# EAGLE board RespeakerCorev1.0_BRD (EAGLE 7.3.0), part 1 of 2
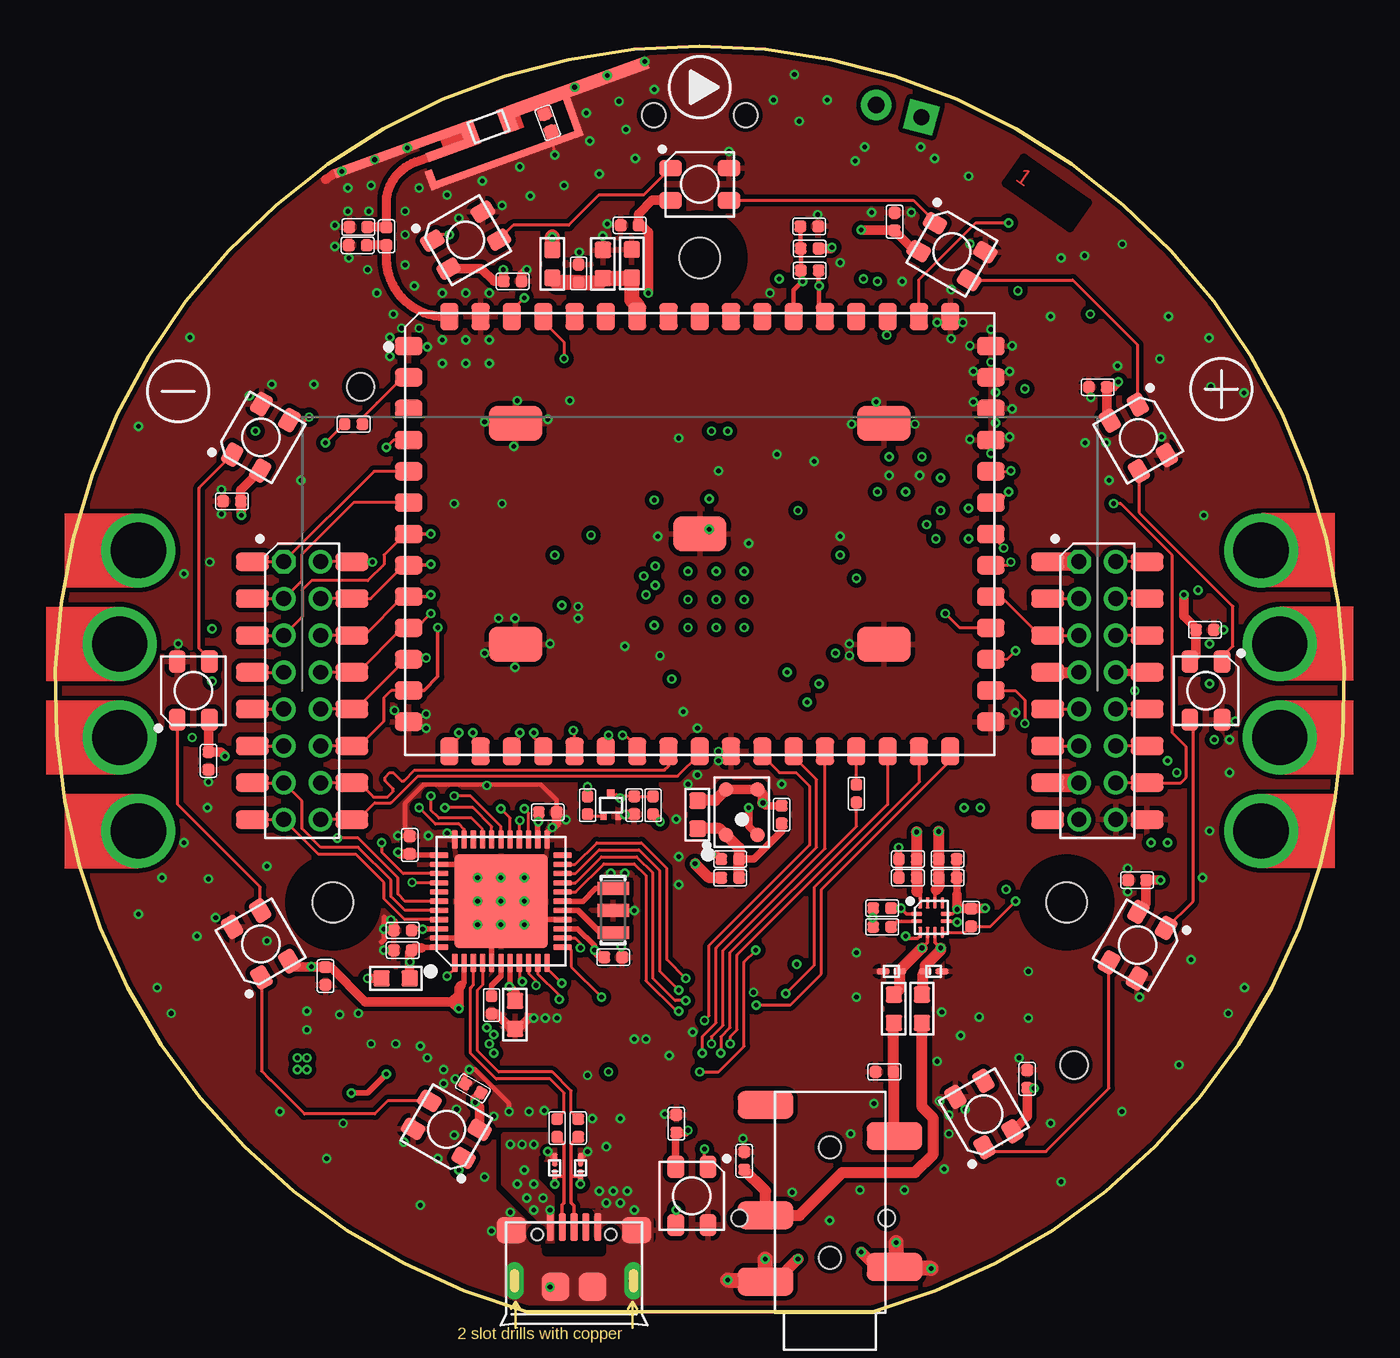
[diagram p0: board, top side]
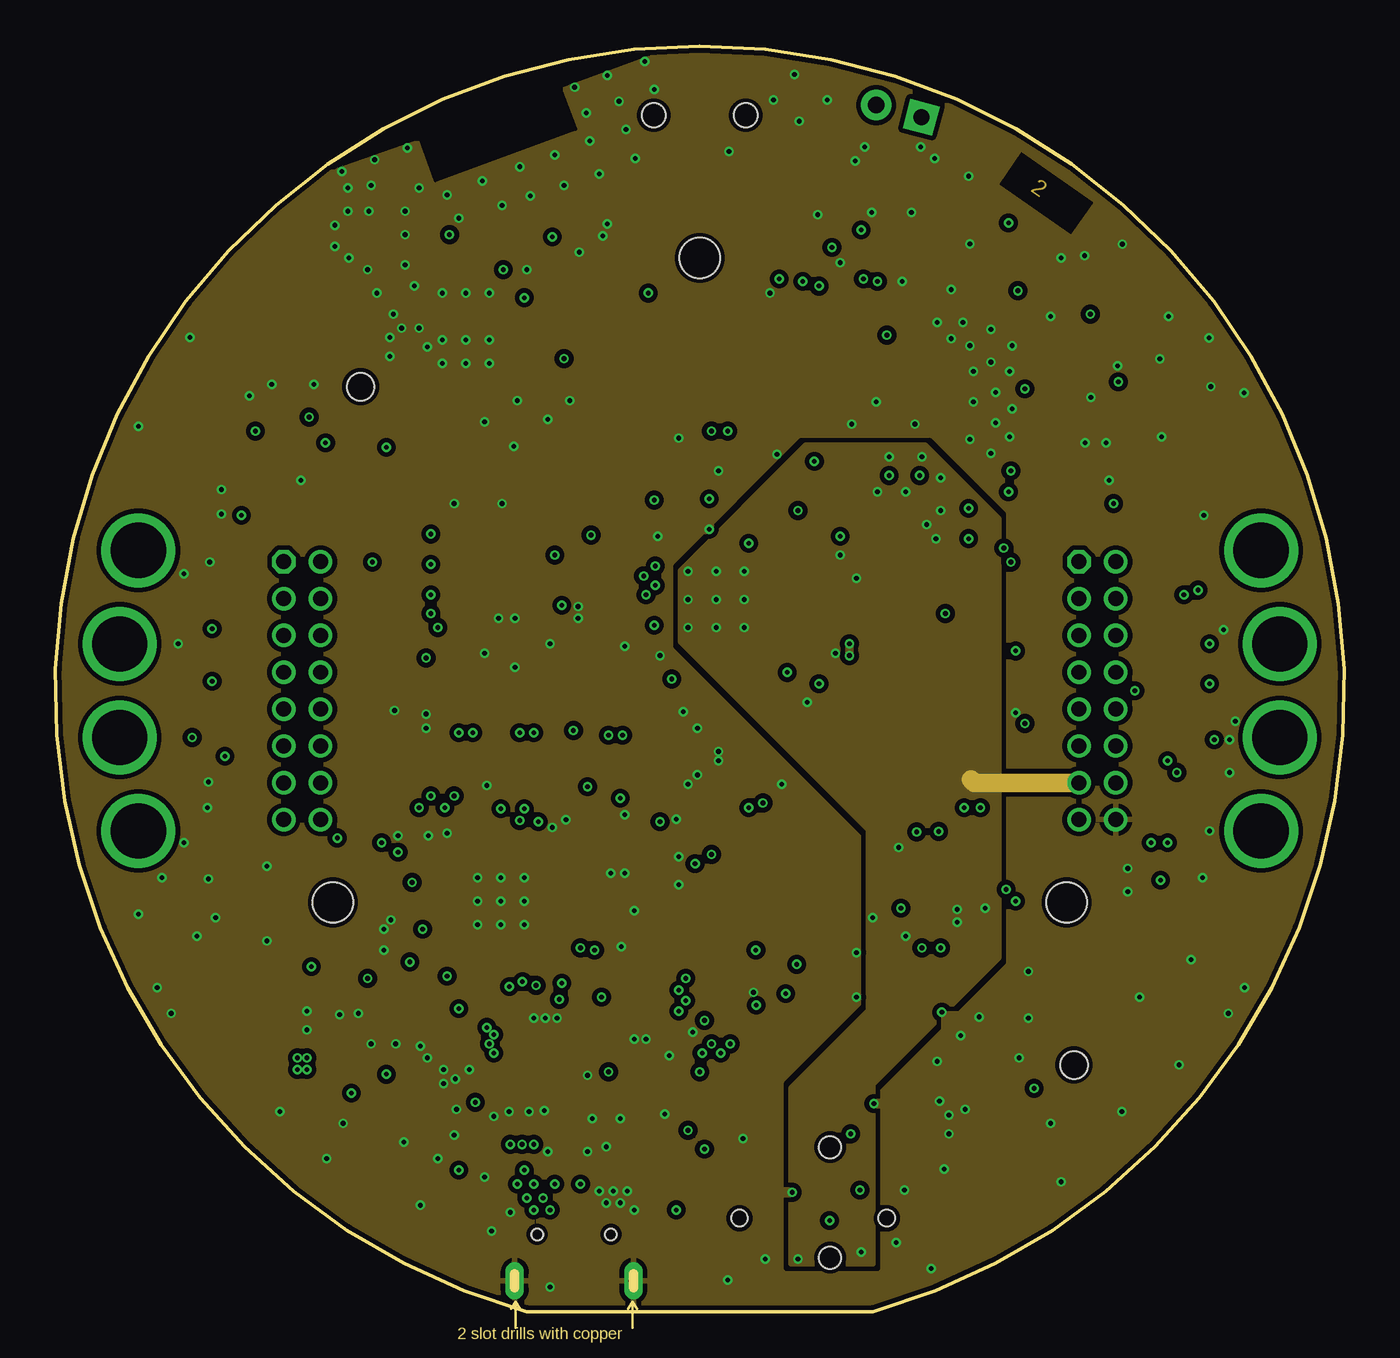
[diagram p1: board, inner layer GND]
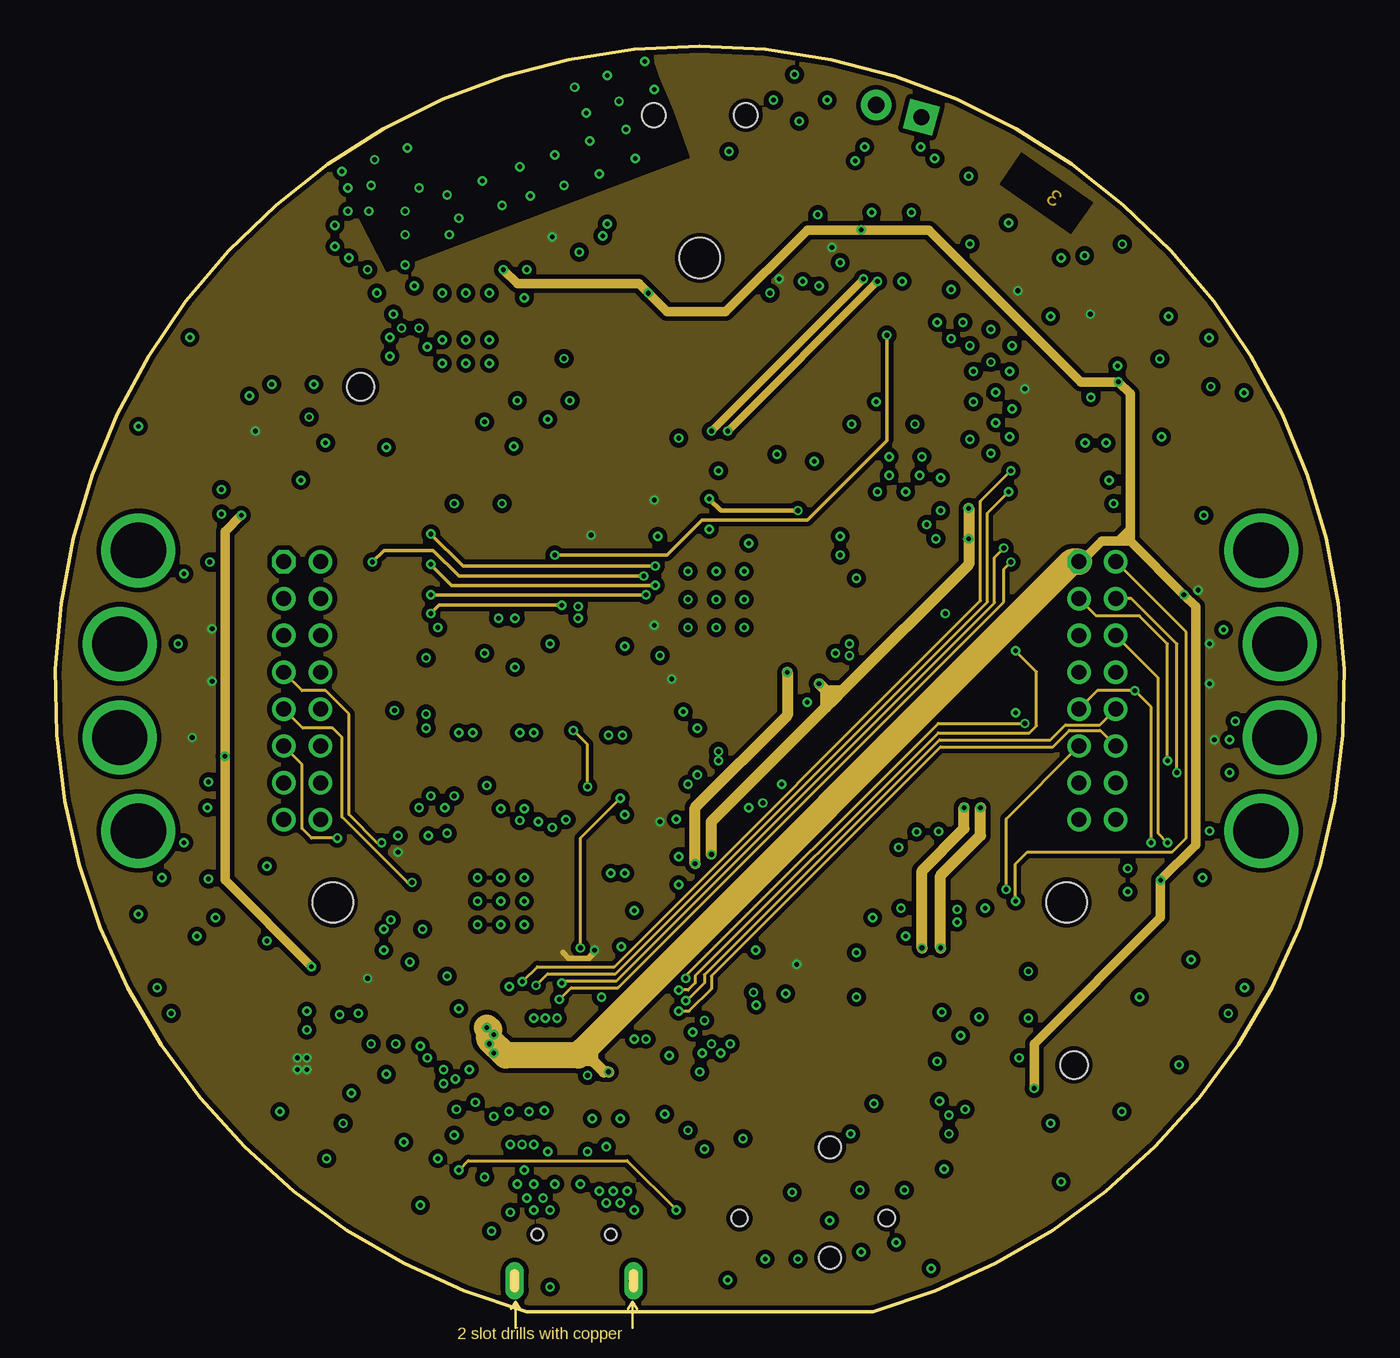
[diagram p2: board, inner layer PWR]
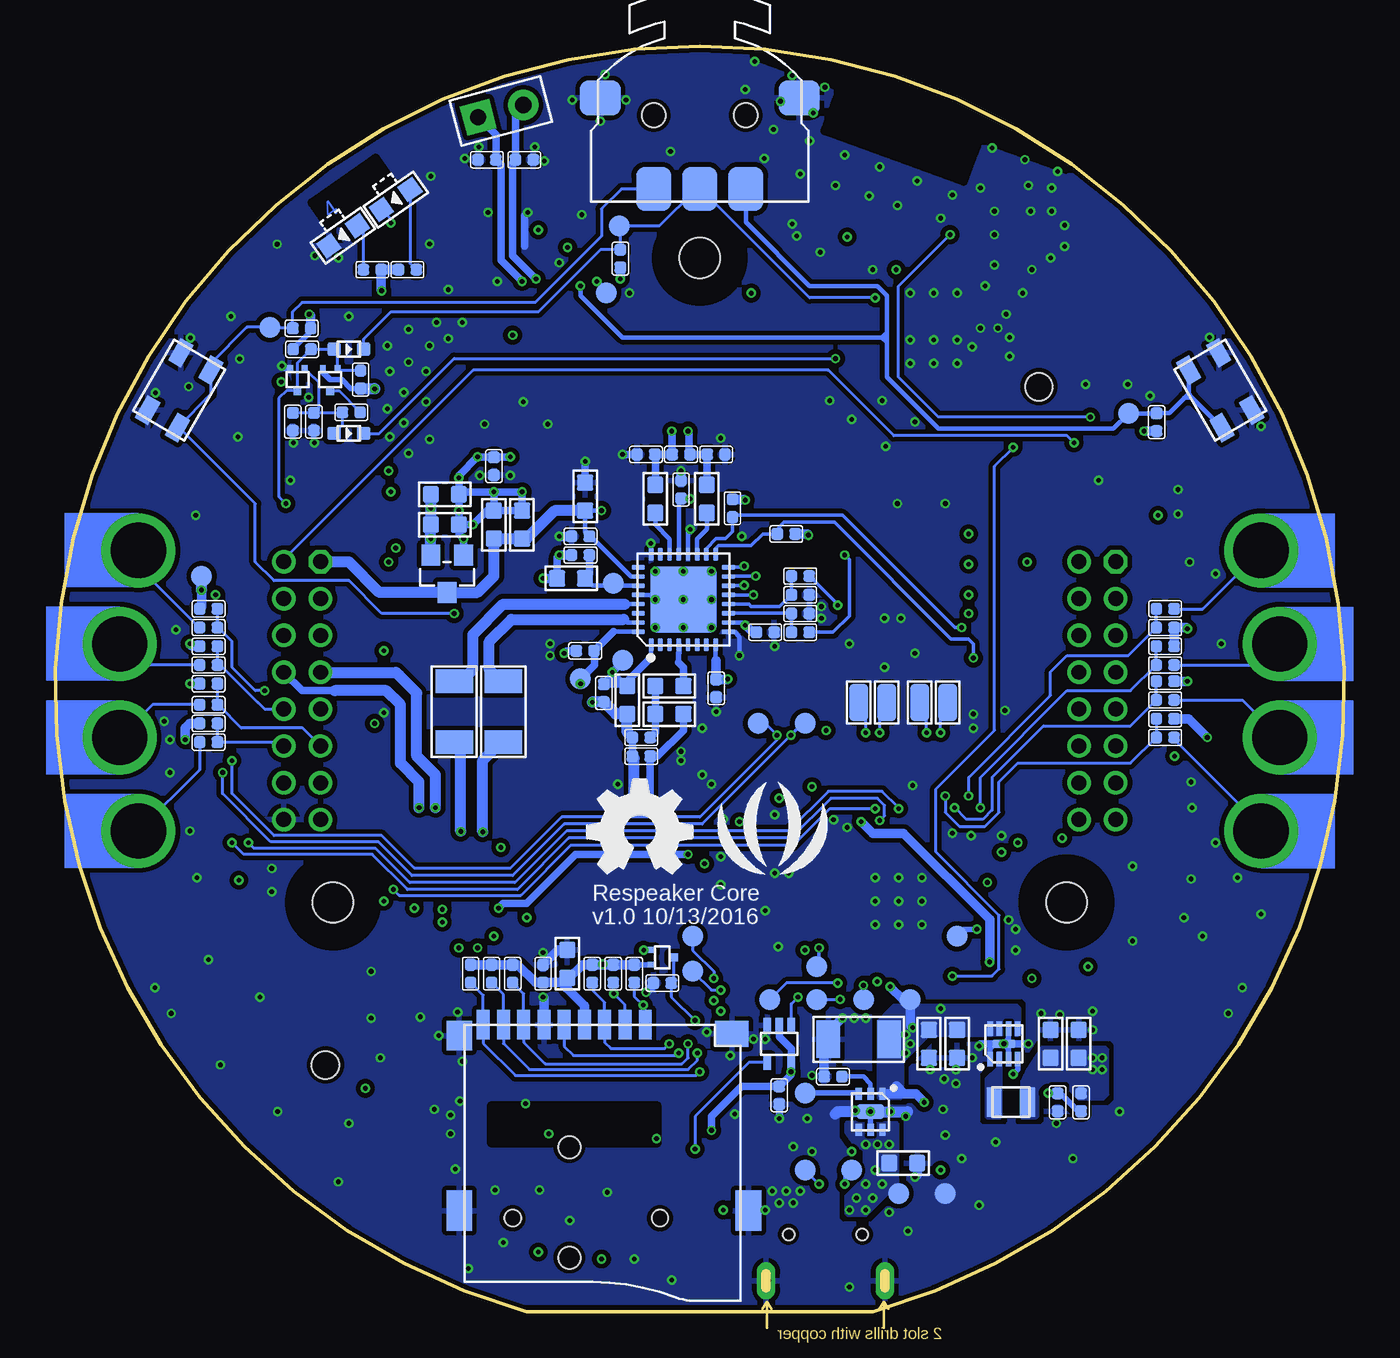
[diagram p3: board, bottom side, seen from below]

Size 69.97 x 68.72 mm. Coordinates in mm from the lower left corner, seen from the top.
Outline: 25.59,0 44.38,0 arc329 25.59,0
Copper layers (1*2*15*16): Top 0.035mm / dielectric 0.2mm / GND 0.0175mm / dielectric 0.3mm / PWR 0.0175mm / dielectric 0.2mm / Bottom 0.035mm
Design rules "SeeedStudio_4layer_DRU_no_angle_20140221 *": minimum track width 1mil, minimum drill 10mil, track to track 6mil, track to pad 6mil, pad to pad 6mil, via to via 6mil, smd to smd 0mil, copper to edge 10mil, drill to drill 8mil, minimum pad ring 6mil, minimum via ring 4mil, stop-mask expansion 4mil, vias tented up to drill 25mil, thermal gap 10mil
Holes 2.2 mm at 15.07,22.22 34.98,57.22 54.9,22.22
Holes 1.5 mm at 16.57,50.23 55.3,13.4
tRestrict: area 32.6,54.9 to 37.3,59.6; area 12.7,19.9 to 17.4,24.6; area 52.6,19.9 to 57.3,24.6; area 51.6,58.9 to 56,62.6
bRestrict: area 32.6,54.9 to 37.3,59.6; area 12.7,19.9 to 17.4,24.6; area 52.6,19.9 to 57.3,24.6; area 51.6,58.9 to 56,62.6; area 17.8,10.7 to 18.2,11.9

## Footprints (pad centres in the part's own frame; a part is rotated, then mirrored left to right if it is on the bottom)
ANT2P-SMD-3.5X1.4MM-BOTTOM = smd 3 x 0.5: ANT -2.5,-0.45 | smd 0.72 x 0.4: C$1 2.8,-0.48; C$2 2.8,-1.32; P$3 2.8,-1.67 | smd 0.8 x 1.4: CHIP1 0.8,0; CHIP2 -1.4,0 | smd 8.4 x 0.4: G$1 0,-2 | smd 0.4 x 2.6: G$2 4.2,-0.9 | smd 0.4 x 1.1: G$4 -4.2,-1.65 | smd 8 x 0.7: GND1 5,0.35 | smd 8 x 0.5: GND2 -5,0.45
BUTTON3+2P-SMD-11.8X11.8X2.5MM = smd 1.9 x 2.4: 1 -2.5,0.7; 2 0,0.7; 3 2.5,0.7 | smd 2.2 x 1.9: 4 5.4,5.65; 5 -5.4,5.65 | hole 1.3: -2.5,4.7; 2.5,4.7
C0402 = smd 0.635 x 0.635: 1 0,0.484; 2 0,-0.484
C0603 = smd 0.889 x 0.889: 1 0,0.762; 2 0,-0.762
C1206 = smd 1.27 x 2.032: 1 -1.651,0; 2 1.651,0
LED4-SMD-3.5X3.7MM = smd 1.2 x 0.9: 1 -1.58,0.875; 2 -1.58,-0.875; 3 1.58,-0.875; 4 1.58,0.875
SOD-923 = smd 0.7 x 0.3: 1 -0.45,0; 2 0.45,0
LED-SIDE-VIEW-0603-RIGHT = smd 1 x 1: 1 0,-0.95; 2 0,0.95
SOD-523 = smd 0.762 x 0.7: + -0.8,0; - 0.8,0
L0603 = smd 0.889 x 0.889: 1 -0.762,0; 2 0.762,0
MICRO-USB5+4P-SMD-0.65-B = smd 0.381 x 1.524: 1 -1.3,-0.25; 2 -0.65,-0.25; 3 0,-0.25; 4 0.65,-0.25; 5 1.3,-0.25 | smd 1.6 x 1.397: S1 -3.4,-0.427; S6 3.4,-0.427 | drill 0.508 pad 1.016 long: S2 -3.226,-3.175; S5 3.226,-3.175 | smd 1.5 x 1.5: S3 -1,-3.5; S4 1,-3.5 | hole 0.635: -2,-0.65; 2,-0.65
AUDIO5P-14X5X4.4MM = smd 3 x 1.5: 2 -3.5,-11.6; 3 -3.5,-4.5; 4 3.5,-3.7; 5 3.5,-7.3; 6 3.5,-13.3 | hole 1.2: 0,-5; 0,-11
1P-DIP-6X4MM = drill 3 pad 4: 1 0,0
H2-2.54 = drill 0.889 pad 1.651 square: 1 0,1.27 | drill 0.889 pad 1.651: 2 0,-1.27
H2X8-SMD_DRILL-2.0 = smd 1.8 x 1: 1 -2.7,7; 2 2.7,7; 3 -2.7,5; 4 2.7,5; 5 -2.7,3; 6 2.7,3; 7 -2.7,1; 8 2.7,1; 9 -2.7,-1; 10 2.7,-1; 11 -2.7,-3; 12 2.7,-3; 13 -2.7,-5; 14 2.7,-5; 15 -2.7,-7; 16 2.7,-7 | drill 0.813 pad 1.27 octagon: P$1 -1,7 | drill 0.813 pad 1.27: P$2 1,7; P$3 -1,5; P$4 1,5; P$5 -1,3; P$6 1,3; P$7 -1,1; P$8 1,1; P$9 -1,-1; P$10 1,-1; P$11 -1,-3; P$12 1,-3; P$13 -1,-5; P$14 1,-5; P$15 -1,-7; P$16 1,-7
MICRO-SD9+4P-SMD-16.1X14.5X1.85MM = smd 1.6 x 0.7: 1 0,2.25; 2 0,1.15; 3 0,0.05; 4 0,-1.05; 5 0,-2.15; 6 0,-3.25; 7 0,-4.35; 8 0,-5.45; 9 0,-6.55 | smd 1.6 x 1.4: G1 0.6,-7.85 | smd 2.2 x 1.4: G2 10.1,-7.85; G3 10.1,7.85 | smd 1.4 x 1.8: G4 0.5,6.95 | hole 0.9: 10.5,-4.95; 10.5,3.05
SW4P-SMD-4.5X3.2X2.5MM = smd 1.4 x 0.8: 1 -1.8,-0.94; 2 1.8,-0.94; 3 1.8,0.94; 4 -1.8,0.94
L201610 = smd 0.8 x 1.6: 1 -0.9,0; 2 0.9,0
R0402 = smd 0.635 x 0.635: 1 0,0.484; 2 0,-0.484
MIC4-SMD-3.76X2.95MM = smd 0.8 x 0.8: 1 0.85,1.23; 2 0.85,-1.23; 3 -0.85,-1.23; 4 -0.85,1.23
SOT-723 = smd 0.32 x 0.4: 1 -0.4,-0.6; 2 0.4,-0.6 | smd 0.42 x 0.5: 3 0,0.6
TP-D45MIL = smd 1.143 x 1.143: T 0,0
TP-80X40MIL = smd 2.032 x 1.016: 1 0,0
DFN6G-0.65-2X2MM = smd 0.65 x 0.35: 1 -0.975,0.65; 2 -0.975,0; 3 -0.975,-0.65; 4 0.975,-0.65; 5 0.975,0; 6 0.975,0.65 | smd 0.8 x 1.5: PAD 0,0
DFN8G-0.5-2X2MM = smd 0.8 x 0.3: 1 -0.827,0.75; 2 -0.827,0.25; 3 -0.827,-0.25; 4 -0.827,-0.75; 5 0.827,-0.75; 6 0.827,-0.25; 7 0.827,0.25; 8 0.827,0.75 | smd 0.45 x 1.3: 9 0,0
SOT-353 = smd 0.4 x 0.8: 1 -0.65,-1; 2 0,-1; 3 0.65,-1; 4 0.65,1; 5 -0.65,1
SOT-23 = smd 1.016 x 1.143: 1 -0.889,-1.016; 2 0.889,-1.016; 3 0,1.016
QFN32G-0.5-5X5MM = smd 0.7 x 0.25: 1 -2.45,1.75; 2 -2.45,1.25; 3 -2.45,0.75; 4 -2.45,0.25; 5 -2.45,-0.25; 6 -2.45,-0.75; 7 -2.45,-1.25; 8 -2.45,-1.75; 17 2.45,-1.75; 18 2.45,-1.25; 19 2.45,-0.75; 20 2.45,-0.25; 21 2.45,0.25; 22 2.45,0.75; 23 2.45,1.25; 24 2.45,1.75 | smd 0.25 x 0.7: 9 -1.75,-2.45; 10 -1.25,-2.45; 11 -0.75,-2.45; 12 -0.25,-2.45; 13 0.25,-2.45; 14 0.75,-2.45; 15 1.25,-2.45; 16 1.75,-2.45; 25 1.75,2.45; 26 1.25,2.45; 27 0.75,2.45; 28 0.25,2.45; 29 -0.25,2.45; 30 -0.75,2.45; 31 -1.25,2.45; 32 -1.75,2.45 | smd 3.6 x 3.6: 33 0,0
LGA65-1.7-24X32X1.8MM = smd 1.5 x 1: 1 -15.8,10.2; 2 -15.8,8.5; 3 -15.8,6.8; 4 -15.8,5.1; 5 -15.8,3.4; 6 -15.8,1.7; 7 -15.8,0; 8 -15.8,-1.7; 9 -15.8,-3.4; 10 -15.8,-5.1; 11 -15.8,-6.8; 12 -15.8,-8.5; 13 -15.8,-10.2; 31 15.8,-10.2; 32 15.8,-8.5; 33 15.8,-6.8; 34 15.8,-5.1; 35 15.8,-3.4; 36 15.8,-1.7; 37 15.8,0; 38 15.8,1.7; 39 15.8,3.4; 40 15.8,5.1; 41 15.8,6.8; 42 15.8,8.5; 43 15.8,10.2 | smd 1 x 1.5: 14 -13.6,-11.8; 15 -11.9,-11.8; 16 -10.2,-11.8; 17 -8.5,-11.8; 18 -6.8,-11.8; 19 -5.1,-11.8; 20 -3.4,-11.8; 21 -1.7,-11.8; 22 0,-11.8; 23 1.7,-11.8; 24 3.4,-11.8; 25 5.1,-11.8; 26 6.8,-11.8; 27 8.5,-11.8; 28 10.2,-11.8; 29 11.9,-11.8; 30 13.6,-11.8; 44 13.6,11.8; 45 11.9,11.8; 46 10.2,11.8; 47 8.5,11.8; 48 6.8,11.8; 49 5.1,11.8; 50 3.4,11.8; 51 1.7,11.8; 52 0,11.8; 53 -1.7,11.8; 54 -3.4,11.8; 55 -5.1,11.8; 56 -6.8,11.8; 57 -8.5,11.8; 58 -10.2,11.8; 59 -11.9,11.8; 60 -13.6,11.8 | smd 2.9 x 1.9: 61 10,6; 62 -10,6; 63 -10,-6; 64 10,-6; 65 0,0
VQFN-44 = smd 1 x 0.3: 1 -3.35,2.5; 2 -3.35,2; 3 -3.35,1.5; 4 -3.35,1; 5 -3.35,0.5; 6 -3.35,0; 7 -3.35,-0.5; 8 -3.35,-1; 9 -3.35,-1.5; 10 -3.35,-2; 11 -3.35,-2.5; 23 3.35,-2.5; 24 3.35,-2; 25 3.35,-1.5; 26 3.35,-1; 27 3.35,-0.5; 28 3.35,0; 29 3.35,0.5; 30 3.35,1; 31 3.35,1.5; 32 3.35,2; 33 3.35,2.5 | smd 0.3 x 1: 12 -2.5,-3.35; 13 -2,-3.35; 14 -1.5,-3.35; 15 -1,-3.35; 16 -0.5,-3.35; 17 0,-3.35; 18 0.5,-3.35; 19 1,-3.35; 20 1.5,-3.35; 21 2,-3.35; 22 2.5,-3.35; 34 2.5,3.35; 35 2,3.35; 36 1.5,3.35; 37 1,3.35; 38 0.5,3.35; 39 0,3.35; 40 -0.5,3.35; 41 -1,3.35; 42 -1.5,3.35; 43 -2,3.35; 44 -2.5,3.35 | smd 5.08 x 5.08: TAB 0,0
LEAD12P-SMD-0.4-1.8X1.8X0.5MM = smd 0.6 x 0.2: 1 -0.8,0.2; 2 -0.8,-0.2; 7 0.8,-0.2; 8 0.8,0.2 | smd 0.2 x 0.6: 3 -0.6,-0.8; 4 -0.2,-0.8; 5 0.2,-0.8; 6 0.6,-0.8; 9 0.6,0.8; 10 0.2,0.8; 11 -0.2,0.8; 12 -0.6,0.8
RESONATOR3-SMD-3.6X1.3X0.8MM = smd 0.7 x 1.7: 1 -1.2,0; 2 0,0; 3 1.2,0

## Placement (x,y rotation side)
ANT1  [ANT2P-SMD-3.5X1.4MM-BOTTOM]  23.8,64.45 20 top
BUTTON1  [BUTTON3+2P-SMD-11.8X11.8X2.5MM]  34.98,60.26 0 bottom
C1  100nF  [C0402]  45.56,59.19 0 top
C2  100nF  [C0402]  31.43,27.5 180 top
C3  100nF  [C0402]  56.59,50.2 90 top
C4  100nF  [C0402]  62.42,37.02 270 top
C5  10uF  [C0603]  23.94,8.06 270 bottom
C6  10uF  [C0603]  21.01,14.54 180 bottom
C7  10uF  [C0603]  22.54,14.54 180 bottom
C8  10uF  [C0603]  14.41,14.54 0 bottom
C9  10uF  [C0603]  15.93,14.54 0 bottom
C10  100uF 10V  [C1206]  26.35,14.8 0 bottom
C11  100nF  [C0402]  58.73,23.43 90 top
C12  100nF  [C0402]  52.76,12.64 0 top
C13  10uF  [C0603]  44.64,42.74 0 bottom
C14  10uF  [C0603]  46.16,42.74 0 bottom
C15  10uF  [C0603]  48.83,42.74 270 bottom
C16  10uF  [C0603]  48.83,44.39 270 bottom
C17  100nF  [C0402]  33.71,10.21 0 top
C18  10uF  [C0603]  34.86,26.99 0 top
C19  100nF  [C0402]  57.08,48.32 180 bottom
C20  33pF  [C0402]  29.52,38.93 270 bottom
C22  100nF  [C0402]  31.43,36.89 270 bottom
C23  100nF  [C0402]  34.1,33.85 180 bottom
C24  100nF  [C0402]  41.21,35.88 90 bottom
C25  100uF 10V  [C1206]  48.32,32.58 270 bottom
C26  100uF 10V  [C1206]  45.65,32.58 270 bottom
C27  100nF  [C0402]  53.4,50.61 0 bottom
C28  100pF  [C0402]  46.29,24.57 90 top
C29  100pF  [C0402]  48.45,24.57 270 top
C31  680nF DNP  [C0402]  36,46.55 90 bottom
C32  100pF  [C0402]  34.1,46.55 270 bottom
C33  100pF  [C0402]  37.91,46.55 90 bottom
C34  100pF  [C0402]  44.51,62.55 270 bottom
C35  100pF  [C0402]  46.54,62.55 90 bottom
C36  10uF  [C0603]  36.64,33.97 90 bottom
C37  100nF  [C0402]  39.43,26.99 0 top
C38  33pF  [C0402]  38.16,30.16 90 bottom
C39  33pF  [C0402]  38.16,31.18 90 bottom
C41  100nF  [C0402]  22.67,12.13 60 top
C42  100nF  [C0402]  14.66,18.22 180 top
C43  100nF  [C0402]  8.31,29.91 180 top
C44  100nF  [C0402]  9.58,44.01 90 top
C45  100nF  [C0402]  24.82,55.94 270 top
C46  100nF  [C0402]  31.17,58.99 90 top
C48  100nF  [C0402]  30.67,11.75 180 bottom
C49  10uF  [C0603]  41.21,44.26 180 bottom
C50  100nF  [C0402]  36,44.64 0 bottom
C51  100nF  [C0402]  41.46,42.1 90 bottom
C52  10uF  [C0603]  38.92,33.21 0 bottom
C53  100nF  [C0402]  40.19,33.59 180 bottom
C54  10uF  [C0603]  41.97,39.81 270 bottom
C55  100nF  [C0402]  41.46,41.08 90 bottom
C56  10uF  [C0603]  42.18,18.88 180 bottom
C57  1uF  [C0402]  43.49,18.35 180 bottom
C58  10uF  [C0603]  29.73,56.88 180 top
C59  10uF  [C0603]  31.29,56.91 180 top
C60  100nF  [C0402]  28.41,56.37 0 top
C61  1uF  [C0402]  40.93,58.93 270 top
C62  1uF  [C0402]  23.68,16.65 180 top
C63  100nF  [C0402]  30.29,19.24 270 top
C64  100nF  [C0402]  19.24,25.34 0 top
C65  100nF  [C0402]  26.73,27.11 270 top
C66  100nF  [C0402]  18.86,19.62 90 top
C67  100nF  [C0402]  18.86,20.7 90 top
C68  100nF  [C0402]  44.89,20.89 90 top
C69  100nF  [C0402]  44.89,21.91 90 top
C71  33pF  [C0402]  37.4,8.19 0 top
C72  33pF  [C0402]  45.02,13.02 90 top
C74  10uF  [C0603]  24.95,16.12 0 top
C75  33pF  [C0402]  29.52,37.91 270 bottom
D1  SK6812  [LED4-SMD-3.5X3.7MM]  48.68,57.56 150 top
D2  SK6812  [LED4-SMD-3.5X3.7MM]  58.8,47.45 120 top
D3  SK6812  [LED4-SMD-3.5X3.7MM]  62.47,33.72 90 top
D4  SK6812  [LED4-SMD-3.5X3.7MM]  58.76,19.9 60 top
D5  SK6812  [LED4-SMD-3.5X3.7MM]  50.42,10.73 300 top
D6  DF2S6.8FS  [SOD-923]  28.51,7.81 90 top
D7  DF2S6.8FS  [SOD-923]  27.11,7.81 90 top
D8  SK6812  [LED4-SMD-3.5X3.7MM]  34.55,6.29 90 top
D9  SK6812  [LED4-SMD-3.5X3.7MM]  21.23,9.9 330 top
D10  SK6812  [LED4-SMD-3.5X3.7MM]  11.15,19.96 300 top
D11  Green  [LED-SIDE-VIEW-0603-RIGHT]  54.35,58.42 125 bottom
D12  Red  [LED-SIDE-VIEW-0603-RIGHT]  51.49,60.39 125 bottom
D13  SK6812  [LED4-SMD-3.5X3.7MM]  7.49,33.72 270 top
D14  SK6812  [LED4-SMD-3.5X3.7MM]  11.15,47.47 240 top
D15  DF2S6.8FS  [SOD-923]  45.4,18.48 180 top
D16  DF2S6.8FS  [SOD-923]  47.68,18.48 0 top
D18  SK6812  [LED4-SMD-3.5X3.7MM]  22.27,58.19 210 top
D19  SK6812  [LED4-SMD-3.5X3.7MM]  34.98,61.22 180 top
D20  1N4148WT  [SOD-523]  54.03,52.26 0 bottom
D21  1N4148WT  [SOD-523]  54.03,47.69 0 bottom
FB1  120R 500mA  [L0603]  26.98,56.9 270 top
FB2  120R-500mA  [L0603]  18.47,18.1 0 top
FR1  [SEEEDSTUDIO-PCB-FRAME]  not placed on the board
FR2  [SEEEDSTUDIO-PCB-FRAME]  not placed on the board
FR3  [SEEEDSTUDIO-PCB-FRAME]  not placed on the board
FR4  [SEEEDSTUDIO-PCB-FRAME]  not placed on the board
FR5  [SEEEDSTUDIO-PCB-FRAME]  not placed on the board
FR7  [SEEEDSTUDIO-PCB-FRAME]  not placed on the board
J1  MICRO-USB  [MICRO-USB5+4P-SMD-0.65-B]  28.16,4.85 0 top
J2  PJ327-327  [AUDIO5P-14X5X4.4MM]  42.06,-2.07 180 top
J3  [1P-DIP-6X4MM]  65.46,41.34 90 top
J4  DNP  [H2-2.54]  45.79,65.19 105 bottom
J5  EH  [H2X8-SMD_DRILL-2.0]  13.39,33.72 0 top
J6  [H2X8-SMD_DRILL-2.0]  56.57,33.72 0 top
J7  [MICRO-SD9+4P-SMD-16.1X14.5X1.85MM]  40.19,15.58 270 bottom
J8  [1P-DIP-6X4MM]  66.48,36.26 90 top
J9  [1P-DIP-6X4MM]  66.48,31.18 90 top
J10  [1P-DIP-6X4MM]  65.46,26.1 90 top
J11  [1P-DIP-6X4MM]  4.5,26.1 270 top
J12  [1P-DIP-6X4MM]  3.49,31.18 270 top
J13  [1P-DIP-6X4MM]  3.49,36.26 270 top
J14  [1P-DIP-6X4MM]  4.5,41.34 270 top
K1  [SW4P-SMD-4.5X3.2X2.5MM]  6.72,50.04 300 bottom
K2  [SW4P-SMD-4.5X3.2X2.5MM]  63.25,50.04 60 bottom
L1  0.47uH  [L201610]  18.09,11.37 0 bottom
L2  BLM18BD252SN1  [L0603]  47.05,16.45 270 top
L4  BLM18BD252SN1  [L0603]  45.53,16.45 270 top
L6  BLM18BD252SN1  [L0603]  37.4,44.13 90 bottom
L7  BLM18BD252SN1  [L0603]  34.6,44.13 90 bottom
L8  BLM18BD252SN1  [L0603]  36.64,32.45 180 bottom
LC1  6.8nH  [R0402]  16.45,58.89 90 top
LC2  1.5pF  [R0402]  16.41,57.9 90 top
LC3  1.6pF  [R0402]  17.98,58.4 0 top
LC4  dnp  [R0402]  26.73,64.55 20 top
MIC1  SAO-3729-M-42-008  [MIC4-SMD-3.76X2.95MM]  37.27,27.11 180 top
Q1  CJ3134K  [SOT-723]  30.16,27.5 0 top
Q2  CJ3139K  [SOT-723]  37.02,19.24 270 bottom
Q3  CJ3139K  [SOT-723]  55.05,50.61 180 bottom
Q4  CJ3134K  [SOT-723]  56.83,50.61 180 bottom
R1  10k  [R0402]  32.44,27.5 0 top
R2  1k  [R0402]  28.89,27.5 180 top
R3  100k_1%  [R0402]  55.94,48.32 0 bottom
R4  10k dnp  [R0402]  56.57,52.26 270 bottom
R5  100k_1%  [R0402]  14.28,11.37 180 bottom
R6  22K_1%  [R0402]  27.75,12.76 90 bottom
R7  22K_1%  [R0402]  15.55,11.37 180 bottom
R8  10M  [R0402]  61.65,31.94 270 bottom
R9  22R  [R0402]  27.24,9.97 0 top
R10  22R  [R0402]  28.38,9.97 0 top
R11  10k  [R0402]  39.29,57.18 0 bottom
R12  1k  [R0402]  52.76,56.58 90 bottom
R13  10M  [R0402]  9.71,32.19 90 bottom
R14  10M  [R0402]  9.71,34.23 90 bottom
R15  10M  [R0402]  9.71,36.13 90 bottom
R16  10M  [R0402]  9.71,37.15 90 bottom
R17  1k  [R0402]  50.86,56.58 270 bottom
R18  33R  [R0402]  9.71,38.16 90 bottom
R19  33R  [R0402]  61.65,30.92 270 bottom
R20  33R  [R0402]  9.71,35.12 90 bottom
R21  33R  [R0402]  9.71,33.21 90 bottom
R22  1k  [R0402]  10.18,48.3 0 bottom
R23  33R  [R0402]  9.71,31.18 90 bottom
R24  10k  [R0402]  47.43,18.35 180 bottom
R25  10k  [R0402]  46.29,18.35 180 bottom
R26  10k  [R0402]  45.14,18.35 180 bottom
R27  10k  [R0402]  40.83,18.35 180 bottom
R28  10k  [R0402]  39.68,18.35 180 bottom
R29  10k  [R0402]  38.54,18.35 180 bottom
R30  10k  [R0402]  46.29,23.56 90 top
R31  10k  [R0402]  48.45,23.56 270 top
R32  22R  [R0402]  43.49,28.13 180 top
R33  10k  [R0402]  56.6,53.4 90 bottom
R34  0R  [R0402]  46.16,45.91 180 bottom
R35  10M  [R0402]  61.65,34.1 270 bottom
R36  33R  [R0402]  61.65,32.96 270 bottom
R37  10M  [R0402]  61.65,36.13 270 bottom
R38  10k  [R0402]  33.21,43.62 180 bottom
R39  10k  [R0402]  30.29,42.23 90 bottom
R40  22R  [R0402]  29.52,39.94 90 bottom
R41  33R  [R0402]  61.65,35.12 270 bottom
R42  10M  [R0402]  61.65,38.16 270 bottom
R43  33R  [R0402]  61.65,37.15 270 bottom
R46  100k_1%  [R0402]  53.91,48.83 270 bottom
R47  2.2k  [R0402]  49.72,21.4 0 top
R48  0R  [R0402]  16.19,48.2 270 top
R49  22R  [R0402]  29.52,36.89 90 bottom
R53  10k  [R0402]  40.95,57.73 90 top
R55  0R DNP  [R0402]  40.96,56.53 90 top
R56  10k  [R0402]  37.02,17.84 90 bottom
R57  0R  [R0402]  36.64,23.56 90 top
R58  0R DNP  [R0402]  36.64,24.57 90 top
TP1  [TP-D45MIL]  23.55,16.95 180 bottom
TP2  [TP-D45MIL]  62.04,39.94 180 bottom
TP3  [TP-D45MIL]  24.19,6.41 180 bottom
TP4  [TP-D45MIL]  41.46,34.35 180 bottom
TP5  [TP-D45MIL]  26.09,16.95 270 bottom
TP6  [TP-D45MIL]  39.35,58.96 158 bottom
TP7  [TP-D45MIL]  28.63,16.95 270 bottom
TP8  [TP-D45MIL]  31.17,16.95 270 bottom
TP9  [TP-80X40MIL]  21.52,33.08 270 bottom
TP10  [TP-80X40MIL]  23.05,33.08 270 bottom
TP11  [TP-80X40MIL]  24.82,33.08 270 bottom
TP12  [TP-D45MIL]  11.69,48.77 60 bottom
TP13  [TP-D45MIL]  39.18,35.37 180 bottom
TP14  [TP-D45MIL]  39.68,39.56 180 bottom
TP15  [TP-D45MIL]  58.33,53.45 188 bottom
TP16  [TP-D45MIL]  29.27,31.94 180 bottom
TP17  [TP-D45MIL]  31.81,31.94 180 bottom
TP18  [TP-D45MIL]  21.65,6.41 0 bottom
TP19  [TP-D45MIL]  26.73,7.68 0 bottom
TP20  [TP-D45MIL]  29.27,7.68 0 bottom
TP21  [TP-D45MIL]  29.27,11.87 0 bottom
TP22  [TP-80X40MIL]  26.35,33.08 270 bottom
TP23  [TP-D45MIL]  28.63,18.73 0 bottom
TP24  [TP-D45MIL]  35.37,18.48 180 bottom
TP25  [TP-D45MIL]  35.37,20.38 180 bottom
TP26  [TP-D45MIL]  40.06,55.31 0 bottom
TP27  [TP-D45MIL]  21.01,20.38 0 bottom
U1  ETA6020  [DFN6G-0.65-2X2MM]  25.71,10.86 270 bottom
U2  ETA3410  [DFN8G-0.5-2X2MM]  18.47,14.54 90 bottom
U3  74HC1G08  [SOT-353]  30.67,14.54 180 bottom
U4  AP7333  [SOT-23]  48.7,40.07 180 bottom
U5  WM8960  [QFN32G-0.5-5X5MM]  35.87,38.67 90 bottom
U6  AI7688H  [LGA65-1.7-24X32X1.8MM]  34.98,42.23 0 top
U7  ATMEGA32U4  [VQFN-44]  24.19,22.29 90 top
U8  FSA2275  [LEAD12P-SMD-0.4-1.8X1.8X0.5MM]  47.56,21.4 0 top
U$75  [OSHW_FILLX200_NOTEXT_TNAME]  41.08,23.81 0 bottom
U$76  [SEEED-SILK-TNAME-280*268MIL]  31.05,25.46 0 bottom
X3  16MHz-16pF-0.5%-40R  [RESONATOR3-SMD-3.6X1.3X0.8MM]  30.29,21.78 270 top

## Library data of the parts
ANT1 J1 J3-J6 J8-J14 MIC1 = Connector-new
BUTTON1 J2 U8 = template
C1-C20 C22-C29 C31-C39 C41-C46 C48-C69 C71 C72 C74 C75 D1-D16 D18-D21 FB1 FB2 K1 K2 L1 L2 L4 L6-L8 LC1-LC4 Q1-Q4 R1-R43 R46-R49 R53 R55-R58 TP9-TP11 TP22 X3 = Discrete-new
FR1-FR5 FR7 U6 = moudle-new
J7 = Connector-new; SKU: 320090000
TP1-TP8 TP12-TP21 TP23-TP27 = Discrete-new; PARTNO: DNP
U1-U5 U7 = IC-new
U$75 U$76 = Logo

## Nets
!PWR_ON: C27.1 D20.+ J6.14 J6.P$14 Q3.1 Q4.3 R4.1
AGND: C13.1 C14.1 C15.1 C16.1 C18.1 C24.1 C28.1 C29.1 C37.1 C38.1 C39.1 C52.2 C53.1 C54.2 C55.1 C68.1 C69.1 J2.3 J2.4 J6.13 J6.P$13 MIC1.2 MIC1.3 R30.1 R31.1 R34.2 R47.1 U4.1 U5.28 U5.33 U8.3 U8.7 U8.8
AVDD: C15.2 C16.2 C24.2 C69.2 R58.1 TP4.T U4.2 U5.32 U8.1
GND: ANT1.G$1 ANT1.G$2 ANT1.G$4 ANT1.GND1 ANT1.GND2 BUTTON1.4 BUTTON1.5 C1.1 C2.1 C3.1 C4.1 C5.1 C6.1 C7.1 C8.1 C9.1 C10.1 C11.1 C12.1 C17.1 C19.1 C20.1 C22.1 C23.1 C32.1 C33.1 C34.1 C35.1 C41.1 C42.1 C43.1 C44.1 C45.1 C46.1 C48.1 C49.2 C50.1 C51.1 C56.2 C57.2 C58.2 C59.2 C60.1 C61.1 C62.1 C63.1 C64.1 C65.1 C66.1 C67.1 C71.1 C72.1 C74.2 C75.1 D1.2 D2.2 D3.2 D4.2 D5.2 D6.2 D7.2 D8.2 D9.2 D10.2 D11.2 D13.2 D14.2 D15.2 D16.2 D18.2 D19.2 J1.5 J1.S1 J1.S2 J1.S3 J1.S4 J1.S5 J1.S6 J6.16 J6.P$16 J7.6 J7.G1 J7.G2 J7.G3 J7.G4 K1.3 K1.4 K2.3 K2.4 LC1.1 LC2.1 LC4.1 LC4.2 Q1.2 Q4.2 R3.2 R6.1 R7.1 R34.1 R56.1 TP18.T U1.5 U1.PAD U2.1 U2.3 U2.6 U2.9 U3.3 U5.9 U5.20 U5.24 U6.1 U6.13 U6.23 U6.31 U6.40 U6.41 U6.42 U6.43 U6.44 U6.59 U6.61 U6.62 U6.63 U6.64 U6.65 U7.5 U7.15 U7.23 U7.33 U7.35 U7.43 U7.TAB X3.2
GPIO12/UART_TXD0: J6.4 J6.P$4 TP16.T U6.19
GPIO13/UART_RXD0: J6.3 J6.P$3 TP17.T U6.20
GPIO_0/I2S_ADC: J5.5 J5.P$5 U5.16 U6.7
GPIO_1/I2S_DAC: J5.4 J5.P$4 U5.14 U6.8
GPIO_2/I2S_LRCLK: J5.6 J5.P$6 U5.13 U6.9
GPIO_3/I2S_BCLK: J5.8 J5.P$8 R40.2 U6.10
GPIO_4/I2C_SCL: J5.10 J5.P$10 R39.1 U5.17 U6.11
GPIO_5/I2C_SDA: J5.12 J5.P$12 R38.1 U5.18 U6.12
GPIO_19/PWM_CH1: BUTTON1.1 K2.1 K2.2 R33.1 TP15.T U6.34
GPIO_40: D21.- U6.57
GPIO_41: R48.1 U6.2
GPIO_42: BUTTON1.2 D20.- R11.1 TP6.T U6.58
GPIO_45/UART_TXD1: J5.1 J5.P$1 U6.5
GPIO_46/UART_RXD1: J5.3 J5.P$3 U6.6
HP_L: D15.1 J6.7 J6.P$7 L4.1 U8.4
HP_R: D16.1 J6.8 J6.P$8 L2.1 U8.5
HP_SEL: J6.2 J6.P$2 R47.2 R48.2 U8.6
LIN1: C36.2 U5.4
MCLK_OUT: J5.2 J5.P$2 U5.15
MIC_VDD: C18.2 C37.2 MIC1.1 R57.2 R58.2
MICBIAS: C52.1 C53.2 R57.1 TP13.T U5.1
MT_GPIO0: R2.2 U6.18
MT_GPIO_14/SPIS_CS: U6.39 U7.8
MT_GPIO_18/PWM_CH0: J6.5 J6.P$5 U6.35
MT_GPIO_39: U6.4 U7.1
MT_GPIO_43: U6.3
MT_SPIS_CLK: TP5.T U6.38 U7.9
MT_SPIS_MISO: TP8.T U6.37 U7.11
MT_SPIS_MOSI: TP7.T U6.36 U7.10
MT_UART_RXD: TP25.T U6.32 U7.21
MT_UART_TXD: TP24.T U6.33 U7.20
N$1: Q3.3 R46.1
N$2: LC2.2 LC3.2 U6.60
N$3: D11.1 R12.1
N$4: C68.2 U8.2
N$5: C75.2 R49.1 U5.11
N$6: C38.2 L8.1 MIC1.4
N$7: D12.1 R17.1
N$8: R10.1 U7.4
N$9: J7.5 R32.1
N$10: R9.1 U7.3
N$11: D9.1 D10.3
N$12: R6.2 U1.2
N$13: D1.3 D19.1
N$14: L6.1 U5.22
N$15: D7.1 J1.2 R9.2 TP19.T
N$16: D6.1 J1.3 R10.2 TP20.T
N$18: D10.1 D13.3
N$19: D8.1 D9.3
N$20: J13.1 R20.2
N$21: C19.2 D21.+ Q4.1 R3.1 R46.2
N$22: J14.1 R18.2
N$23: D13.1 D14.3
N$24: C36.1 C39.2 L8.2
N$25: D14.1 D18.3
N$26: C20.2 R40.1 U5.12
N$27: TP9.1 U6.14
N$28: Q1.1 R2.1
N$29: L1.1 U2.2
N$30: D18.1 D19.3
N$31: J8.1 R41.2
N$32: R5.1 R7.2 U2.4
N$33: J12.1 R21.2
N$34: J11.1 R23.2
N$35: J3.1 R43.2
N$36: J9.1 R36.2
N$37: J10.1 R19.2
N$38: L7.1 U5.19
N$39: C31.1 C33.2 C35.2 J4.1 L6.2
N$40: C62.2 U7.6
N$41: C67.2 TP27.T U7.42
N$42: D1.1 D2.3
N$43 [none3]: C65.2 C66.2 FB2.2 U7.24 U7.44
N$44: D2.1 D3.3
N$45: D3.1 D4.3
N$46: D4.1 D5.3
N$47: C31.2 C32.2 C34.2 J4.2 L7.2
N$49: U7.17 X3.1
N$50: U7.16 X3.3
N$51: ANT1.ANT LC1.2 LC3.1
N$52: TP10.1 U6.15
N$53: TP11.1 U6.16
N$54: TP22.1 U6.17
N$57: C26.2 C28.2 R30.2 U8.12
N$58: C25.1 U5.29
N$59: D8.3 U3.4
N$60: C26.1 U5.31
N$61: C25.2 C29.2 R31.2 U8.10
N$63: C72.2 J2.2 L4.2
N$64: C71.2 J2.5 L2.2
PB4/A8/D8: R13.1 R23.1 U7.28
PB5/A9/D9: R14.1 R21.1 U7.29
PB6/A10/D10: R16.1 R18.1 U7.30
PB7/D11: U3.1 U7.12
PC7/D13: R15.1 R20.1 U7.32
PD0/SCL/D3: J6.12 J6.P$12 R8.1 R19.1 U7.18
PD1/SDA/D2: J6.10 J6.P$10 R37.1 R41.1 U7.19
PD4/A6/D4: J6.11 J6.P$11 R35.1 R36.1 U7.25
PD6/A11/D12: J6.6 J6.P$6 U7.26
PD7/A7/D6: J6.9 J6.P$9 R42.1 R43.1 U7.27
PF0/A5: J5.15 J5.P$15 U7.41
PF1/A4: J5.13 J5.P$13 U7.40
PF4/A3: J5.11 J5.P$11 U7.39
PF6/A1: J5.9 J5.P$9 U7.37
PF7/A0: J5.7 J5.P$7 U7.36
PORST_N: C61.2 R53.1 R55.1 TP26.T U6.49
PW_FAULT: TP21.T U1.3
REF_CLKO: R49.2 U6.46
RIN1: U5.5
RST_A: C2.2 Q1.3 R1.1 TP23.T U7.13
SD_CD: Q2.3 R56.2 U6.24
SD_CLK: R32.2 U6.27
SD_CMD: J7.3 R27.1 U6.28
SD_D0: J7.7 R26.1 U6.26
SD_D1: J7.8 R25.1 U6.25
SD_D2: J7.1 R29.1 U6.30
SD_D3: J7.2 R28.1 U6.29
SSSS: J7.9 Q2.1 R24.1
USB_5V: C5.2 J1.1 TP3.T U1.4 U1.6
USB_M: J5.16 J5.P$16 U6.22
USB_P: J5.14 J5.P$14 U6.21
VDD_3V3: C8.2 C9.2 C22.2 C23.2 C27.2 C56.1 C57.1 C63.2 C64.2 FB1.1 FB2.1 J7.4 L1.2 Q2.2 Q3.2 R1.2 R4.2 R5.2 R8.2 R11.2 R12.2 R13.2 R14.2 R15.2 R16.2 R17.2 R22.2 R24.2 R25.2 R26.2 R27.2 R28.2 R29.2 R33.2 R35.2 R37.2 R38.2 R39.2 R42.2 R53.2 TP2.T U5.8 U5.10 U7.14 U7.34
VDD_5V: C1.2 C3.2 C4.2 C6.2 C7.2 C10.2 C11.2 C12.2 C13.2 C14.2 C17.2 C41.2 C42.2 C43.2 C44.2 C45.2 C46.2 C48.2 C49.1 C50.2 C51.2 C74.1 D1.4 D2.4 D3.4 D4.4 D5.4 D8.4 D9.4 D10.4 D13.4 D14.4 D18.4 D19.4 J6.1 J6.P$1 TP1.T U1.1 U2.5 U2.7 U2.8 U3.2 U3.5 U4.3 U5.21 U5.26 U7.2 U7.7
VDD_7688: C58.1 C59.1 C60.2 FB1.2 U6.54
VMID: C54.1 C55.2 TP14.T U5.27
WDT_RST_N: BUTTON1.3 K1.1 K1.2 R22.1 R55.2 TP12.T U6.48
WLED_N: D12.2 U6.45

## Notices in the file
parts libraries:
moudle-new: This work is licensed under the Creative Commons Attribution 4.0 International License.
To view a copy of this license,visit:
http://creativecommons.org/licenses/by-sa/4.0
